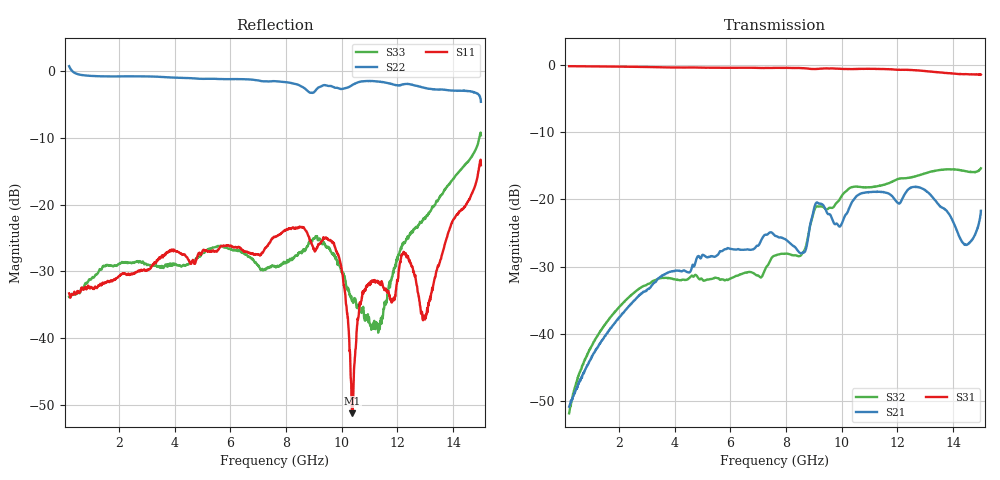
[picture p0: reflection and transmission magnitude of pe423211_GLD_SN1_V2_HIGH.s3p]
! Created Mon Jan 20 11:13:59 2025
# mhz S ri R 50
! 3 Port Network Data from SP1.SP block
! freq  reS11  imS11  reS12  imS12  reS13  imS13
!  reS21  imS21
!  reS22  imS22  reS23  imS23
!  reS31  imS31  reS32  imS32
!  reS33  imS33
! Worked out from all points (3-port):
!   1481 points, 200 MHz to 15 GHz, reference 50 ohm
!   strongest paths, dB at 200 MHz, 3.9 GHz, 7.6 GHz, 11.3 GHz, 15 GHz:
!     S31: -0.2, -0.4, -0.5, -0.6, -1.5
!     S21: -50.8, -30.7, -25.4, -18.9, -21.7
!     S32: -51.8, -31.8, -28.3, -18.0, -15.4
!   lowest |S11| = -51.2 dB at 10.38 GHz (marker M1), VSWR 1.01, Z = 49.8 - j0.147 ohm
!   |S11| at or under -10 dB: start of sweep to end of sweep
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200  0.0217 -0.000958  0.00287 -0.000399  0.9732 -0.0333
     0.00287 -0.000376  -0.4194 -1  0.00176 0.00201
     0.9734 -0.0333  0.00169 0.00196  0.0204 0.00158
770  0.0224 0.00884  0.00197 -0.00504  0.9625 -0.1294
     0.00206 -0.00498  -0.9072 -0.1804  0.00263 0.00596
     0.9631 -0.1294  0.00267 0.00595  0.0244 0.00701
2200  0.0238 0.0193  -0.00738 -0.0129  0.8968 -0.3566
      -0.00736 -0.0129  -0.8455 0.3377  0.00724 0.016
      0.897 -0.3568  0.00732 0.016  0.0348 0.0123
7600  0.0502 -0.0276  -0.0298 0.0448  0.2637 -0.9094
      -0.0298 0.0447  -0.0185 0.8374  0.0158 0.0348
      0.2632 -0.9088  0.0158 0.0349  0.0323 0.0124
9710  0.0401 -0.0311  -0.0103 0.0662  -0.0893 -0.9337
      -0.0103 0.0663  0.3139 0.6864  0.0399 0.0785
      -0.0894 -0.933  0.04 0.0784  0.0414 0.00753
10380  -0.00232 -0.00147  -0.0325 0.0909  -0.195 -0.9073
       -0.0325 0.0909  0.3173 0.7176  0.0848 0.0898
       -0.1949 -0.9068  0.0849 0.0898  0.0115 -0.0153
10820  -0.0117 0.0195  -0.00224 0.1122  -0.2679 -0.8916
       -0.00214 0.1123  0.409 0.7313  0.1004 0.0704
       -0.2682 -0.8919  0.1006 0.0705  -0.00517 -0.0128
12250  -0.0426 -0.0101  0.0404 0.1002  -0.4926 -0.7726
       0.0403 0.1002  0.5268 0.597  0.1392 0.0337
       -0.4925 -0.7722  0.1394 0.0336  0.00102 0.0518
12970  -0.00396 0.014  0.0909 0.0751  -0.5893 -0.6788
       0.091 0.0752  0.6011 0.4452  0.1555 0.00627
       -0.5889 -0.6779  0.1554 0.00613  0.00373 0.0778
15000  -0.0691 0.1847  0.00837 0.082  -0.7168 -0.4449
       0.00831 0.0819  0.5442 0.2208  0.1112 -0.1293
       -0.716 -0.4447  0.1109 -0.1289  -0.1429 0.2973
